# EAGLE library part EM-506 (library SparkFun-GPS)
USGlobalSat EM-506 High Performance GPS Module EM-506 GPS module features high sensitivity, low power and ultra small form factor. This GPS module is powered by SiRF Star IV, it can provide you with superior sensitivity and performance even in urban canyon and dense foliage environment. With SiRF CGEE (Client Generated Extended Ephemeris) technology, it predicts satellite positions for up to 3 days and delivers CGEE-start time of less than 15 seconds under most conditions, without any network assistance. Besides, MicroPower Mode allows GPS module to stay in a hot-start condition nearly continuously while consuming very little power. SparkFun Products GPS Receiver - EM-506 (48 Channel) (GPS-12751)
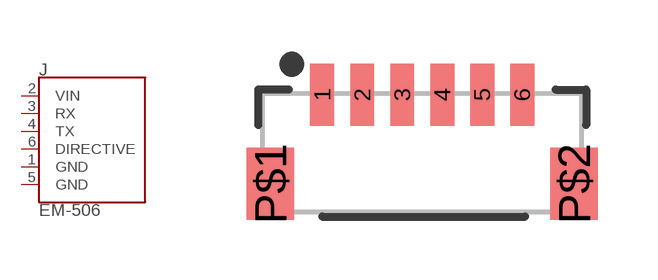
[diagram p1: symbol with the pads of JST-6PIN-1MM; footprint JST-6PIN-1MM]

Designator prefix J

## EM-506-VERTICAL (PROD_ID: CONN-08249)  [JST-6PIN-1MM]
1  GND
2  VIN
3  RX
4  TX
5  GND
6  DIRECTIVE

## Footprint JST-6PIN-1MM (pad centres in mm)
6-Pin Vertical JST Connector 1.0mm pitch JST-SH type Common interface for SparkFun GPS modules. Datasheet
smd 0.6 x 1.55: 1 -2.5,1.45; 2 -1.5,1.45; 3 -0.5,1.45; 4 0.5,1.45; 5 1.5,1.45; 6 2.5,1.45
smd 1.2 x 1.8: P$1 -3.8,-0.775; P$2 3.8,-0.775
